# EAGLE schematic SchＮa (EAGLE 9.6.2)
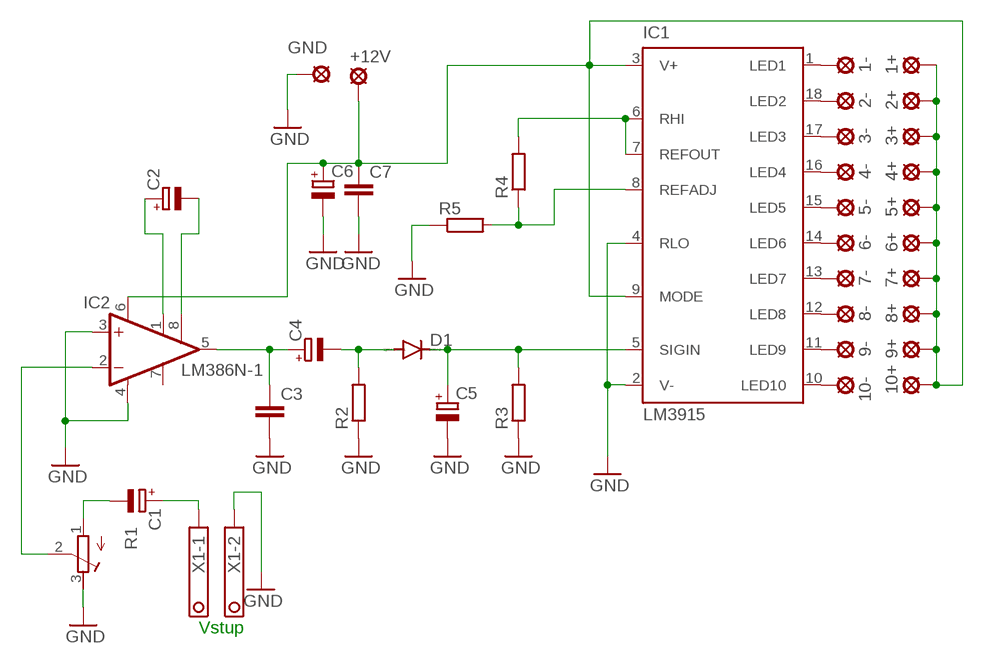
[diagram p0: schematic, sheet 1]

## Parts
1+  MCS10B  [MCS10B]
1-  MCS10B  [MCS10B]
2+  MCS10B  [MCS10B]
2-  MCS10B  [MCS10B]
3+  MCS10B  [MCS10B]
3-  MCS10B  [MCS10B]
4+  MCS10B  [MCS10B]
4-  MCS10B  [MCS10B]
5+  MCS10B  [MCS10B]
5-  MCS10B  [MCS10B]
6+  MCS10B  [MCS10B]
6-  MCS10B  [MCS10B]
7+  MCS10B  [MCS10B]
7-  MCS10B  [MCS10B]
8+  MCS10B  [MCS10B]
8-  MCS10B  [MCS10B]
9+  MCS10B  [MCS10B]
9-  MCS10B  [MCS10B]
10+  MCS10B  [MCS10B]
10-  MCS10B  [MCS10B]
+12V  MCS08  [MCS08]
C1  CPOL-EUE2.5-5  [E2,5-5]
C2  CPOL-EUE2.5-5  [E2,5-5]
C3  C-EU050-030X075  [C050-030X075]
C4  CPOL-EUE2.5-5  [E2,5-5]
C5  CPOL-EUE2.5-5  [E2,5-5]
C6  CPOL-EUE2.5-5  [E2,5-5]
C7  C-EU050-030X075  [C050-030X075]
D1  1N4148DO35-7  [DO35-7]
GND  MCS08  [MCS08]
IC1  LM3915  LM3914N  [DIL18]
IC2  LM386N-1  [DIL08]
R1  R-TRIMM74W  [RTRIM74W]
R2  R-EU_0204/7  [0204/7]
R3  R-EU_0204/7  [0204/7]
R4  R-EU_0204/7  [0204/7]
R5  R-EU_0204/7  [0204/7]
X1  1751248  [1751248]

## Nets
GND: C3.2 C5.- C6.- C7.2 GND.MP IC1.2(V-) IC1.4(RLO) IC2.3(+IN) IC2.4(GND) R1.3(E) R2.1 R3.1 R5.1 X1.2
N$1: C2.+ IC2.1(GAIN)
N$2: C2.- IC2.8(GAIN)
N$3: C3.1 C4.+ IC2.5(OUT)
N$4: C4.- D1.A R2.2
N$5: C5.+ D1.C IC1.5(SIGIN) R3.2
N$6: IC2.2(-IN) R1.2(S)
N$7: C1.- R1.1(A)
N$8: C1.+ X1.1
N$10: IC1.8(REFADJ) R4.1 R5.2
N$11: IC1.6(RHI) IC1.7(REFOUT) R4.2
N$12: 1+.MP 2+.MP 3+.MP 4+.MP 5+.MP 6+.MP 7+.MP 8+.MP 9+.MP 10+.MP +12V.MP C6.+ C7.1 IC1.3(V+) IC1.9(MODE) IC2.6(VS)
N$13: 1-.MP IC1.1(LED1)
N$14: 2-.MP IC1.18(LED2)
N$15: 3-.MP IC1.17(LED3)
N$16: 4-.MP IC1.16(LED4)
N$17: 5-.MP IC1.15(LED5)
N$18: 6-.MP IC1.14(LED6)
N$19: 7-.MP IC1.13(LED7)
N$20: 8-.MP IC1.12(LED8)
N$21: 9-.MP IC1.11(LED9)
N$22: 10-.MP IC1.10(LED10)
Unconnected: IC2.7(BYPASS)

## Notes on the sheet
- Vstup

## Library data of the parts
1+ 1- 2+ 2- 3+ 3- 4+ 4- 5+ 5- 6+ 6- 7+ 7- 8+ 8- 9+ 9- 10+ 10- = solpad:MCS10B: SOLDER PAD
+12V GND = solpad:MCS08: SOLDER PAD
C1 C2 C4-C6 = rcl:CPOL-EU: POLARIZED CAPACITOR, European symbol; SPICEPREFIX: C
C3 C7 = rcl:C-EU: CAPACITOR, European symbol; SPICEPREFIX: C
D1 = diode:1N4148: DIODE
IC1 = national-semiconductor:LM391: Dot/Bar Display Driver Source: Data sheet LM3915 Data sheet LM3914
IC2 = linear:LM386?-*: Low Voltage Audio Power Amplifier Source: http://cache.national.com/ds/LM/LM386.pdf
R1 = rcl:R-TRIMM: Trimm resistor; SPICEMODEL: X; SPICEPREFIXL: POT
R2-R5 = rcl:R-EU_: RESISTOR, European symbol; SPICEPREFIX: R
X1 = con-phoenix-350:1751248: MKDS 1/ 2-3,5 Printklemme; OC_FARNELL: unknown; OC_NEWARK: unknown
